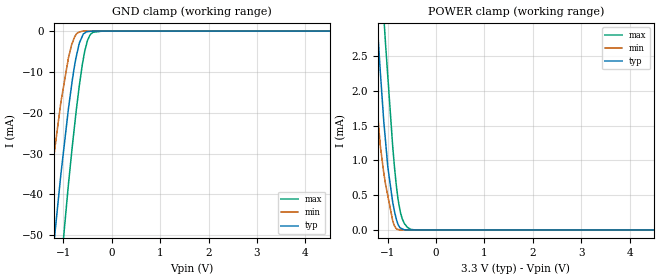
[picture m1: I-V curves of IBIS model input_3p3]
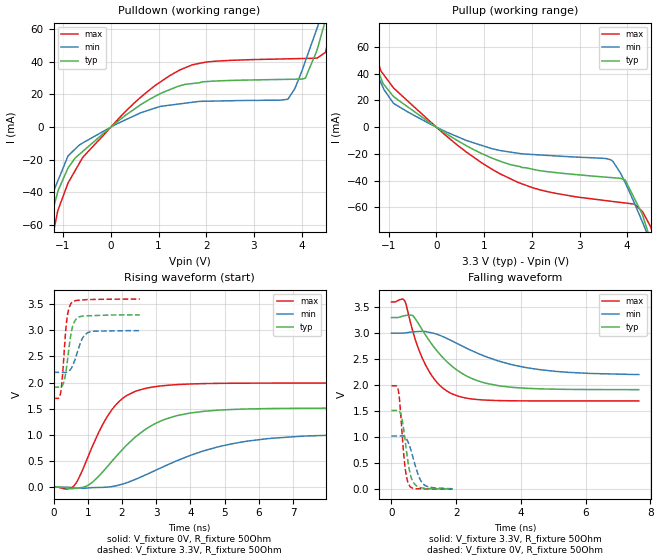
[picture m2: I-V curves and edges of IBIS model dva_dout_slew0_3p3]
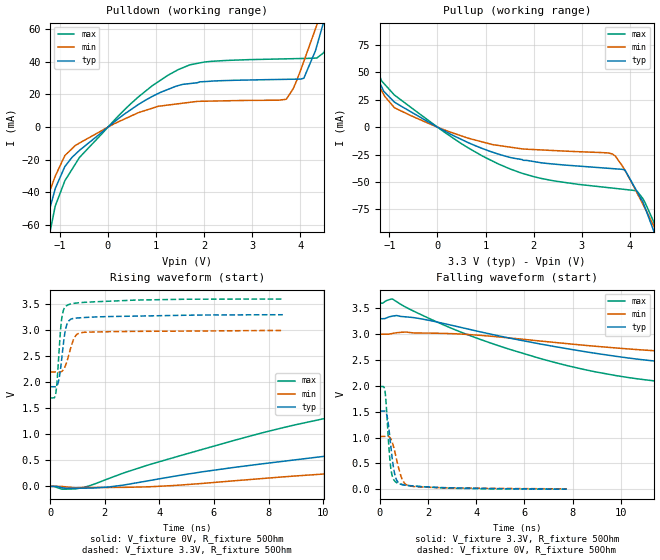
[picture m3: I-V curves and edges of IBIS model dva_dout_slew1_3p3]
|Texas Instruments Incorporated
| 32 Channel Current-Input 20-bit ADC
| Marketing part#   Digital Voltage Range   Package-type   #pins
| DDC232CGXGR   2.0V-3.6V   NFBGA   64
| DDC232CGXGT   2.0V-3.6V   NFBGA   64
| DDC232CKZXGR   2.0V-3.6V   NFBGA   64
| DDC232CKZXGT   2.0V-3.6V   NFBGA   64
| DDC232CZXGR   2.0V-3.6V   NFBGA   64
| DDC232CZXGT   2.0V-3.6V   NFBGA   64
[IBIS Ver]   4.1
[File name]   ddc232.ibs
[File Rev]   1.0
[Date]   2/19/2013
[Source]
| Texas Instruments Incorporated.
| Analog-eLab Design Center, HPA
| 12500 TI Blvd
| Dallas, TX -75243
[Notes]   Revision History:
| Rev 1.0: 2/19/2013
| - Initial version of the model
| - Model generated from simulations in TISPICE
| - Model matched to SPICE simulation
| - C_comp although listed in numerical order of value are
|   obtained from varying PVT conditions. For PVT conditions for
|   each specific value refer the buffer description under
|   respective [Model]. IBIS model user is responsible for using
|   appropriate C_comp to simulate for Signal Integrity.
[Disclaimer]
| This model is designed as an aid for customers of Texas Instruments.
| TI and its licensors and suppliers make no warranties, either expressed
| or implied, with respect to this  model, including the warranties of
| merchantability or fitness for a particular purpose. The model is
| provided solely on an "as is" basis. The entire risk as to its quality
| and performance is with the customer.
[Copyright]
(C) Copyright 2013 Texas Instruments Incorporated.All rights reserved.
|   DDC232GXG
[Component]   DDC232GXG
[Manufacturer]   TI
[Package]   |64 NFBGA  - GXG package
|   typ   min   max
R_pkg   NA   NA   NA
L_pkg   NA   NA   NA
C_pkg   NA   NA   NA
[Pin]  signal_name   model_name   R_pin   L_pin   C_pin
A1   IN28   nc   NA   NA   NA
A2   IN12   nc   NA   NA   NA
A3   IN32   nc   NA   NA   NA
A4   IN16   nc   NA   NA   NA
A5   AGND   gnd   NA   NA   NA
A6   VREF   nc   NA   NA   NA
A7   DGND   gnd   NA   NA   NA
A8   CONV   input_3p3   NA   NA   NA
B1   IN27   nc   NA   NA   NA
B2   IN11   nc   NA   NA   NA
B3   IN31   nc   NA   NA   NA
B4   IN15   nc   NA   NA   NA
B5   AGND   gnd   NA   NA   NA
B6   VREF   nc   NA   NA   NA
B7   DVDD   power   NA   NA   NA
B8   DIN   input_3p3   NA   NA   NA
C1   IN26   nc   NA   NA   NA
C2   IN10   nc   NA   NA   NA
C3   IN30   nc   NA   NA   NA
C4   IN14   nc   NA   NA   NA
C5   AGND   gnd   NA   NA   NA
C6   DGND   gnd   NA   NA   NA
C7   _RESET   input_3p3   NA   NA   NA
C8   DGND   gnd   NA   NA   NA
D1   IN25   nc   NA   NA   NA
D2   IN9   nc   NA   NA   NA
D3   IN29   nc   NA   NA   NA
D4   IN13   nc   NA   NA   NA
D5   AGND   gnd   NA   NA   NA
D6   AGND   gnd   NA   NA   NA
D7   DGND   gnd   NA   NA   NA
D8   DOUT   dva_dout   NA   NA   NA
E1   IN24   nc   NA   NA   NA
E2   IN8   nc   NA   NA   NA
E3   IN20   nc   NA   NA   NA
E4   IN4   nc   NA   NA   NA
E5   AGND   gnd   NA   NA   NA
E6   AVDD   power   NA   NA   NA
E7   DGND   gnd   NA   NA   NA
E8   NC   nc   NA   NA   NA
F1   IN23   nc   NA   NA   NA
F2   IN7   nc   NA   NA   NA
F3   IN19   nc   NA   NA   NA
F4   IN3   nc   NA   NA   NA
F5   AGND   gnd   NA   NA   NA
F6   AVDD   power   NA   NA   NA
F7   CLK_CFG   input_3p3   NA   NA   NA
F8   CLK   input_3p3   NA   NA   NA
G1   IN22   nc   NA   NA   NA
G2   IN6   nc   NA   NA   NA
G3   IN18   nc   NA   NA   NA
G4   IN2   nc   NA   NA   NA
G5   AGND   gnd   NA   NA   NA
G6   AVDD   power   NA   NA   NA
G7   DIN_CFG   input_3p3   NA   NA   NA
G8   DGND   gnd   NA   NA   NA
H1   IN21   nc   NA   NA   NA
H2   IN5   nc   NA   NA   NA
H3   IN17   nc   NA   NA   NA
H4   IN1   nc   NA   NA   NA
H5   QGND   gnd   NA   NA   NA
H6   AGND   gnd   NA   NA   NA
H7   _DVALID   dva_dout   NA   NA   NA
H8   DCLK   input_3p3   NA   NA   NA
|   DDC232ZXG
[Component]   DDC232ZXG
[Manufacturer]   TI
[Package]   |64 NFBGA  - ZXG package
|   typ   min   max
R_pkg   NA   NA   NA
L_pkg   NA   NA   NA
C_pkg   NA   NA   NA
[Pin]  signal_name   model_name   R_pin   L_pin   C_pin
A1   IN28   nc   NA   NA   NA
A2   IN12   nc   NA   NA   NA
A3   IN32   nc   NA   NA   NA
A4   IN16   nc   NA   NA   NA
A5   AGND   gnd   NA   NA   NA
A6   VREF   nc   NA   NA   NA
A7   DGND   gnd   NA   NA   NA
A8   CONV   input_3p3   NA   NA   NA
B1   IN27   nc   NA   NA   NA
B2   IN11   nc   NA   NA   NA
B3   IN31   nc   NA   NA   NA
B4   IN15   nc   NA   NA   NA
B5   AGND   gnd   NA   NA   NA
B6   VREF   nc   NA   NA   NA
B7   DVDD   power   NA   NA   NA
B8   DIN   input_3p3   NA   NA   NA
C1   IN26   nc   NA   NA   NA
C2   IN10   nc   NA   NA   NA
C3   IN30   nc   NA   NA   NA
C4   IN14   nc   NA   NA   NA
C5   AGND   gnd   NA   NA   NA
C6   DGND   gnd   NA   NA   NA
C7   _RESET   input_3p3   NA   NA   NA
C8   DGND   gnd   NA   NA   NA
D1   IN25   nc   NA   NA   NA
D2   IN9   nc   NA   NA   NA
D3   IN29   nc   NA   NA   NA
D4   IN13   nc   NA   NA   NA
D5   AGND   gnd   NA   NA   NA
D6   AGND   gnd   NA   NA   NA
D7   DGND   gnd   NA   NA   NA
D8   DOUT   dva_dout   NA   NA   NA
E1   IN24   nc   NA   NA   NA
E2   IN8   nc   NA   NA   NA
E3   IN20   nc   NA   NA   NA
E4   IN4   nc   NA   NA   NA
E5   AGND   gnd   NA   NA   NA
E6   AVDD   power   NA   NA   NA
E7   DGND   gnd   NA   NA   NA
E8   NC   nc   NA   NA   NA
F1   IN23   nc   NA   NA   NA
F2   IN7   nc   NA   NA   NA
F3   IN19   nc   NA   NA   NA
F4   IN3   nc   NA   NA   NA
F5   AGND   gnd   NA   NA   NA
F6   AVDD   power   NA   NA   NA
F7   CLK_CFG   input_3p3   NA   NA   NA
F8   CLK   input_3p3   NA   NA   NA
G1   IN22   nc   NA   NA   NA
G2   IN6   nc   NA   NA   NA
G3   IN18   nc   NA   NA   NA
G4   IN2   nc   NA   NA   NA
G5   AGND   gnd   NA   NA   NA
G6   AVDD   power   NA   NA   NA
G7   DIN_CFG   input_3p3   NA   NA   NA
G8   DGND   gnd   NA   NA   NA
H1   IN21   nc   NA   NA   NA
H2   IN5   nc   NA   NA   NA
H3   IN17   nc   NA   NA   NA
H4   IN1   nc   NA   NA   NA
H5   QGND   gnd   NA   NA   NA
H6   AGND   gnd   NA   NA   NA
H7   _DVALID   dva_dout   NA   NA   NA
H8   DCLK   input_3p3   NA   NA   NA
|   Model Selectors
[Model Selector] dva_dout
dva_dout_slew0_3p3  3.3V digital output for slew pin connected to GND
dva_dout_slew1_3p3  3.3V digital output for slew pin connected to VDD
| Models and submodels in the file (3): input_3p3 (Input), dva_dout_slew0_3p3 (Output), dva_dout_slew1_3p3 (Output)
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|   input_3p3 Model
[Model]   input_3p3
Model_type   Input
Vinl = 0.66
Vinh = 2.64
|   typ   min   max
|   (nom PVT)   (fast PVT)   (slow PVT)
C_comp   1.230e-12   1.069e-12   1.397e-12
[Model spec]
|subparameter
Vinl   0.66   0.6   0.72
Vinh   2.64   2.4   2.88
| Where nom  PVT is Nominal Process, 3.3V, 40C
|   Fast PVT is Strong Process,  3.6V, 85C
|   Slow PVT is Weak Process,   3V, 0C
[Voltage Range]   3.3   3   3.6
|Junction Temperature
[Temperature Range]   40   85   0
[Power Clamp Reference]   3.3   3   3.6
[GND Clamp Reference]   0   0   0
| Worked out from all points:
|   GND clamp passes 1 mA (typ) near -0.60 V on its own axis
|   POWER clamp passes 1 mA (typ) near -1.01 V on its own axis
[GND Clamp]
|   Voltage   I(typ)   I(min)   I(max)
-3.3V     -356.6mA   -308.4mA   -394.1mA
-1.431V   -81.56mA   -54.68mA   -109.8mA
-1.21V    -53.35mA   -31.51mA   -77.98mA
-1.05V    -34.69mA   -17.15mA   -57.27mA
-897mV    -18.94mA   -6.516mA   -37.41mA
-782.1mV  -9.25mA    -1.782mA   -24.35mA
-708mV    -4.778mA   -416.2uA   -16.72mA
-673.2mV  -2.948mA   -267.5uA   -13.38mA
-558mV    -445.9uA   -7.09uA    -4.77mA
-504mV    -129.6uA   -1.29uA    -2.311mA
-392.4mV  -5.581uA   -30.99nA   -308.3uA
6.6V      0A         0A         0A
[POWER Clamp]
|   Voltage   I(typ)   I(min)   I(max)
-3.3V     29.71mA    29.56mA    30.41mA
-1.346V   4.523mA    3.137mA    6.194mA
-1.242V   3.295mA    1.97mA     4.941mA
-1.195V   2.738mA    1.567mA    4.386mA
-1.079V   1.548mA    812.5uA    3.06mA
-1.044V   1.274mA    657.4uA    2.674mA
-996.6mV  903.3uA    488.9uA    2.202mA
-896.4mV  401.8uA    133.4uA    1.206mA
-792mV    90.79uA    6.401uA    475.1uA
-655.2mV  2.392uA    319.1nA    93.35uA
-439.2mV  284.4nA    0A         1.038uA
6.6V      0A         0A         0A
|   dva_dout_slew0_3p3 Model
[Model]   dva_dout_slew0_3p3
Model_type   Output
Polarity   Non-Inverting
Vmeas = 1.65
Vref = 0
Cref = 9pF
Rref = 100
|   typ   min   max
|   (nom PVT)   (fast PVT)   (slow PVT)
C_comp   1.352e-12   1.129e-12   1.593e-12
| Where nom  PVT is Nominal Process, 3.3V, 40C
|   Fast PVT is Strong Process,  3.6V, 0C
|   Slow PVT is Weak Process,   3V, 85C
[Voltage Range]   3.3   3   3.6
|Junction Temperature
[Temperature Range]   40   85   0
[Pullup Reference]   3.3   3   3.6
[Pulldown Reference]   0   0   0
[Power Clamp Reference]   3.3   3   3.6
[GND Clamp Reference]   0   0   0
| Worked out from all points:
|   slope of the pulldown table from 0 to 0.495 V, typ, clamps not added: 44.7 ohm
|   slope of the pullup table from 0 to 0.495 V, typ, clamps not added: 44.5 ohm
|   falling waveform, V_fixture 3.3V, R_fixture 50Ohm: 20-80 % time 1.29ns typ, 2.05ns min, 792ps max; typ from 3.3 V to 1.91 V
|   rising waveform, V_fixture 0V, R_fixture 50Ohm: 20-80 % time 1.51ns typ, 2.54ns min, 954ps max; typ from 0 V to 1.51 V
|   rising waveform, V_fixture 3.3V, R_fixture 50Ohm: 20-80 % time 180ps typ, 255ps min, 137ps max; typ from 1.91 V to 3.3 V
|   falling waveform, V_fixture 0V, R_fixture 50Ohm: 20-80 % time 213ps typ, 301ps min, 158ps max; typ from 1.51 V to 0.003 V
[Pulldown]
|   Voltage   I(typ)   I(min)   I(max)
-3.3V     -303.9mA   -224.6mA   -420.8mA
-1.536V   -87.19mA   -65.73mA   -117.7mA
-1.35V    -65.39mA   -50.07mA   -85.82mA
-745.8mV  -18.86mA   -13.37mA   -26.55mA
478.8mV   10.75mA    6.777mA    14.43mA
1.447V    25.26mA    14.24mA    34.98mA
3.711V    29.26mA    17.16mA    41.81mA
4.075V    29.94mA    40.25mA    42.04mA
4.324V    47.38mA    60.67mA    42.26mA
4.468V    62.3mA     72.66mA    45.16mA
4.872V    103.7mA    103mA      92.53mA
6.6V      188.8mA    169.2mA    214mA
[Pullup]
|   Voltage   I(typ)   I(min)   I(max)
-3.3V     157.6mA    144.1mA    174.9mA
-1.71V    87.25mA    75.57mA    103mA
-1.119V   32.73mA    29.79mA    39.99mA
-897mV    22.83mA    17.76mA    29.29mA
633.6mV   -14.02mA   -10.03mA   -18.75mA
1.706V    -29.19mA   -19.5mA    -41.26mA
3.657V    -37.71mA   -24.46mA   -55.43mA
3.957V    -39.5mA    -41.57mA   -56.73mA
4.162V    -54.15mA   -57.83mA   -57.84mA
4.324V    -66.02mA   -71.4mA    -63.39mA
4.468V    -82.3mA    -83.88mA   -73.05mA
6.6V      -347.2mA   -279mA     -432.9mA
[Ramp]
R_load = 50
|   typ   min   max
dV/dt_r   0.907969/1.50558e-09   0.613253/2.53585e-09   1.19482/9.53834e-10
dV/dt_f   0.831897/1.28463e-09   0.481824/2.08301e-09   1.14201/7.92356e-10
[Falling Waveform]
V_fixture = 3.3V
V_fixture_min = 3V
V_fixture_max = 3.6V
R_fixture = 50Ohm
|   Time   V(typ)   V(min)   V(max)
0s        3.3V       3V         3.6V
411ps     3.337V     3.004V     3.621V
655ps     3.339V     3.024V     3.047V
843ps     3.175V     3.033V     2.687V
1.058ns   2.96V      3.031V     2.384V
1.502ns   2.59V      2.957V     1.991V
1.979ns   2.311V     2.817V     1.807V
2.884ns   2.043V     2.557V     1.714V
4.155ns   1.94V      2.338V     1.698V
7.642ns   1.914V     2.205V     1.697V
[Rising Waveform]
V_fixture = 0V
V_fixture_min = 0V
V_fixture_max = 0V
R_fixture = 50Ohm
|   Time   V(typ)   V(min)   V(max)
0s        1.18nV     1.337nV    1.103nV
374ps     -16.39mV   101uV      -37.75mV
599ps     -23.19mV   -10.07mV   26.87mV
1.114ns   82.67mV    -8.995mV   748mV
1.716ns   503.1mV    12.72mV    1.49V
2.138ns   805.2mV    85.38mV    1.753V
2.754ns   1.135V     253.4mV    1.899V
4.029ns   1.422V     614.9mV    1.975V
6.388ns   1.505V     936.4mV    1.991V
15ns      1.513V     1.022V     1.991V
[Rising Waveform]
V_fixture = 3.3V
V_fixture_min = 3V
V_fixture_max = 3.6V
R_fixture = 50Ohm
|   Time   V(typ)   V(min)   V(max)
0s        1.914V     2.197V     1.697V
203ps     1.913V     2.197V     1.787V
249ps     1.932V     2.197V     2.031V
302ps     2.013V     2.196V     2.495V
381ps     2.295V     2.198V     3.162V
525ps     2.983V     2.281V     3.525V
670ps     3.222V     2.526V     3.572V
837ps     3.272V     2.837V     3.581V
994ps     3.279V     2.954V     3.588V
2.522ns   3.297V     2.994V     3.598V
[Falling Waveform]
V_fixture = 0V
V_fixture_min = 0V
V_fixture_max = 0V
R_fixture = 50Ohm
|   Time   V(typ)   V(min)   V(max)
0s        1.512V     1.022V     1.989V
211ps     1.512V     1.023V     1.905V
249ps     1.496V     1.024V     1.725V
298ps     1.425V     1.025V     1.342V
412ps     988mV      1.006V     467.2mV
478ps     671.9mV    954mV      204.4mV
559ps     353.5mV    835.2mV    65.79mV
693ps     115.9mV    549mV      17.07mV
978ps     20.56mV    100.9mV    5.402mV
1.899ns   3.092mV    9.886mV    615.2uV
|   dva_dout_slew1_3p3 Model
[Model]   dva_dout_slew1_3p3
Model_type   Output
Polarity   Non-Inverting
Vmeas = 1.65
Vref = 0
Cref = 9pF
Rref = 100
|   typ   min   max
|   (nom PVT)   (fast PVT)   (slow PVT)
C_comp   1.252e-12   1.014e-12   1.508e-12
| Where nom  PVT is Nominal Process, 3.3V, 40C
|   Fast PVT is Strong Process,  3.6V, 0C
|   Slow PVT is Weak Process,   3V, 85C
[Voltage Range]   3.3   3   3.6
|Junction Temperature
[Temperature Range]   40   85   0
[Pullup Reference]   3.3   3   3.6
[Pulldown Reference]   0   0   0
[Power Clamp Reference]   3.3   3   3.6
[GND Clamp Reference]   0   0   0
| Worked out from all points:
|   slope of the pulldown table from 0 to 0.495 V, typ, clamps not added: 44.7 ohm
|   slope of the pullup table from 0 to 0.495 V, typ, clamps not added: 44.5 ohm
|   falling waveform, V_fixture 3.3V, R_fixture 50Ohm: 20-80 % time 16.1ns typ, 26.8ns min, 9.28ns max; typ from 3.3 V to 1.91 V
|   rising waveform, V_fixture 0V, R_fixture 50Ohm: 20-80 % time 18.1ns typ, 30.3ns min, 10.1ns max; typ from 0 V to 1.51 V
|   rising waveform, V_fixture 3.3V, R_fixture 50Ohm: 20-80 % time 202ps typ, 283ps min, 161ps max; typ from 1.91 V to 3.3 V
|   falling waveform, V_fixture 0V, R_fixture 50Ohm: 20-80 % time 245ps typ, 339ps min, 187ps max; typ from 1.51 V to 0.004 V
[Pulldown]
|   Voltage   I(typ)   I(min)   I(max)
-3.3V     -303.8mA   -224.6mA   -420.7mA
-1.539V   -87.39mA   -65.93mA   -118mA
-1.339V   -63.99mA   -49.37mA   -83.72mA
-745.8mV  -18.45mA   -13.08mA   -25.75mA
478.8mV   10.75mA    6.788mA    14.43mA
1.469V    25.49mA    14.33mA    35.29mA
3.711V    29.26mA    17.16mA    41.81mA
4.075V    29.94mA    40.25mA    42.04mA
4.349V    49.98mA    62.76mA    42.33mA
4.468V    62.3mA     72.66mA    45.08mA
4.736V    90.32mA    92.81mA    75.33mA
6.6V      188.8mA    172.3mA    214mA
[Pullup]
|   Voltage   I(typ)   I(min)   I(max)
-3.3V     157.6mA    144.1mA    174.9mA
-2.094V   114.8mA    100.3mA    133.5mA
-1.71V    87.25mA    75.57mA    103mA
-1.119V   32.73mA    29.79mA    39.99mA
-897.6mV  22.85mA    17.79mA    29.32mA
489.6mV   -11.02mA   -7.862mA   -14.82mA
1.505V    -27.53mA   -18.18mA   -38.01mA
3.642V    -37.81mA   -24.51mA   -55.57mA
3.904V    -39.27mA   -39.61mA   -56.82mA
4.162V    -59.48mA   -60.77mA   -58.79mA
4.507V    -95.64mA   -90.66mA   -87.31mA
6.6V      -359.2mA   -283.8mA   -447.7mA
[Ramp]
R_load = 50
|   typ   min   max
dV/dt_r   0.907486/1.80303e-08   0.608654/3.0314e-08   1.19432/1.00438e-08
dV/dt_f   0.831759/1.59834e-08   0.479937/2.66988e-08   1.14201/9.28037e-09
[Falling Waveform]
V_fixture = 3.3V
V_fixture_min = 3V
V_fixture_max = 3.6V
R_fixture = 50Ohm
|   Time   V(typ)   V(min)   V(max)
0s        3.3V       3V         3.6V
529ps     3.35V      3.016V     3.679V
2.118ns   3.261V     3.021V     3.289V
4.156ns   3.047V     2.978V     2.901V
8.935ns   2.631V     2.767V     2.272V
13.09ns   2.405V     2.633V     2.009V
19.24ns   2.219V     2.534V     1.816V
29.32ns   2.04V      2.408V     1.72V
41.4ns    1.956V     2.304V     1.7V
100ns     1.914V     2.2V       1.697V
[Rising Waveform]
V_fixture = 0V
V_fixture_min = 0V
V_fixture_max = 0V
R_fixture = 50Ohm
|   Time   V(typ)   V(min)   V(max)
0s        1.037nV    1.174nV    976.2pV
1.201ns   -35.04mV   -22.2mV    -24.24mV
6.745ns   364.7mV    107.1mV    883.8mV
11.04ns   639mV      270.7mV    1.398V
15.2ns    875.5mV    375.8mV    1.685V
20.54ns   1.106V     480.4mV    1.859V
30.38ns   1.343V     682.8mV    1.958V
41.53ns   1.449V     834.5mV    1.984V
63.64ns   1.503V     965.9mV    1.99V
100ns     1.512V     1.014V     1.991V
[Rising Waveform]
V_fixture = 3.3V
V_fixture_min = 3V
V_fixture_max = 3.6V
R_fixture = 50Ohm
|   Time   V(typ)   V(min)   V(max)
0s        1.914V     2.197V     1.697V
191ps     1.914V     2.197V     1.756V
295ps     1.999V     2.196V     2.369V
380ps     2.273V     2.199V     3.027V
438ps     2.541V     2.215V     3.287V
539ps     2.96V      2.297V     3.441V
647ps     3.152V     2.464V     3.486V
884ps     3.229V     2.856V     3.516V
1.109ns   3.238V     2.95V      3.529V
8.525ns   3.296V     2.993V     3.597V
[Falling Waveform]
V_fixture = 0V
V_fixture_min = 0V
V_fixture_max = 0V
R_fixture = 50Ohm
|   Time   V(typ)   V(min)   V(max)
0s        1.512V     1.022V     1.989V
202ps     1.513V     1.022V     1.931V
296ps     1.431V     1.024V     1.414V
374ps     1.185V     1.018V     832.2mV
458ps     825.9mV    973.8mV    401.9mV
582ps     378.5mV    801.6mV    182.2mV
737ps     148.1mV    492.4mV    117.2mV
1.005ns   82.15mV    128.3mV    84.16mV
1.42ns    60.12mV    51.71mV    62.75mV
7.751ns   4.203mV    8.772mV    2.173mV
